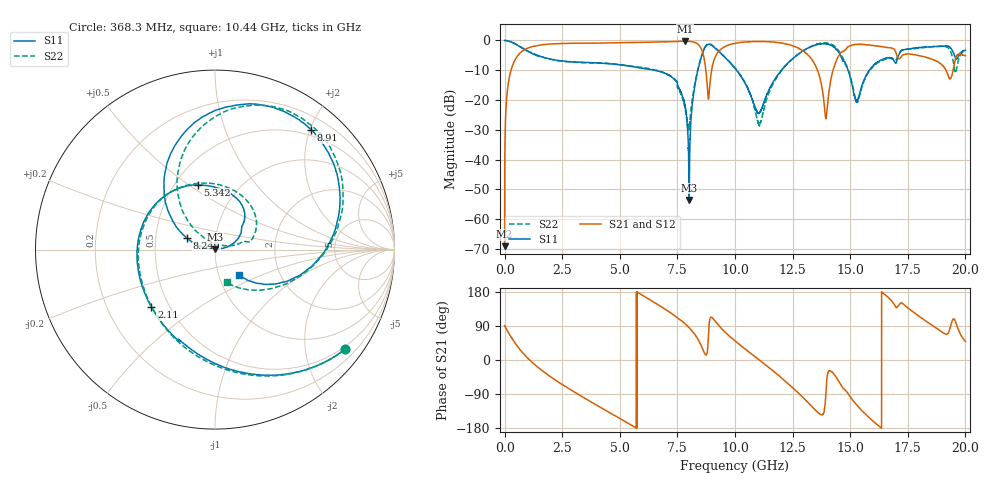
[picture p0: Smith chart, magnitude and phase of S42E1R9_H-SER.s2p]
!{S42E1R9}
!Johanson Technology Inc.
!www.johansontechnology.com
!Test Board Conditions:
!Substrate Type  RO4350B
!Substrate Thickness  50 mil
!Substrate Dk  3.66
!TL Type: GCPW
!TL Trace Width  60 mil
!TL Gap  10 mil
!Electrode orientation  Horizontal
!DUT TOPOLOGY	SERIES
!Mounting Pad LxW  14x55 mil
! Created Wed Nov 25 21:37:39 2020
# khz S ma R 50
! 2 Port Network Data from SP1.SP block
! freq  magS11  angS11  magS21  angS21  magS12  angS12  magS22  angS22
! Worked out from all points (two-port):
!   20001 points, 300 kHz to 20 GHz, reference 50 ohm
!   highest |S21| = -0.25 dB at 7.831 GHz (marker M1); lowest = -69.1 dB at 300 kHz (marker M2)
!   |S21| within 3 dB of the highest: 831.7 MHz to 8.56 GHz (7.729 GHz wide, 165 % of centre); 9.344 GHz to 12.91 GHz (3.565 GHz wide, 32 % of centre)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
!   lowest |S11| = -53.6 dB at 8.009 GHz (marker M3), VSWR 1.00, Z = 50 + j0.209 ohm
!   |S11| at or under -10 dB: 6.507 GHz to 8.388 GHz (1.881 GHz wide, 25.3 % of centre); 10.06 GHz to 12.01 GHz (1.949 GHz wide, 17.7 % of centre); 14.91 GHz to 15.83 GHz (926.2 MHz wide, 6.03 % of centre)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
!   |S22| runs from -30.1 to 0.0 dB; largest |S21 - S12| = 0.017
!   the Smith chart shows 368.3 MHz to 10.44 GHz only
!   S11 on the Smith chart (normalised r, x): 368.3 MHz: 0.43, -2.88; 2.11 GHz: 0.40, -0.33; 5.342 GHz: 0.65, +0.54; 8.249 GHz: 0.72, +0.10; 8.91 GHz: 0.40, +2.02; 10.44 GHz: 1.25, -0.36
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300  0.9996 -0.2  0.0003518 90.4  0.0003525 97.4  1 -0.2
117300  0.989 -12.4  0.14 77.3  0.1402 77.3  0.9895 -12.4
368300  0.9124 -37.6  0.4018 52.8  0.4034 52.8  0.9135 -37.5
2110300  0.4775 -137.9  0.8765 -49.0  0.8765 -49.0  0.4705 -140.3
3334300  0.4305 172.3  0.9002 -95.7  0.8997 -95.7  0.4249 175.8
5342300  0.3736 105.1  0.9178 -166.2  0.9193 -166.4  0.3787 102.3
6667300  0.3055 65.2  0.943 145.5  0.9415 145.4  0.3101 47.9
7831300  0.07897 14.0  0.9717 95.6  0.9709 95.8  0.07275 16.6
8009300  0.002095 86.0  0.9644 85.3  0.9643 85.5  0.03485 92.0
8249300  0.169 157.8  0.9285 68.1  0.9291 68.1  0.1833 134.9
8910300  0.8561 51.2  0.1835 108.4  0.184 108.5  0.8727 48.1
1.00003e7  0.3403 -34.6  0.8948 50.4  0.8949 50.6  0.3444 -40.7
1.04383e7  0.1909 -46.4  0.9416 28.9  0.9416 29.0  0.1949 -69.7
1.10723e7  0.0618 11.4  0.961 -1.0  0.9606 -0.8  0.03882 169.4
1.23283e7  0.4276 27.1  0.8522 -63.6  0.8554 -63.3  0.4265 22.1
1.33343e7  0.7969 -30.1  0.4782 -122.7  0.4831 -122.9  0.8035 -41.1
1.39443e7  0.8761 -79.6  0.04894 -88.1  0.04871 -88.4  0.9089 -85.3
1.44743e7  0.6525 -130.4  0.5275 -52.9  0.5284 -53.1  0.6938 -130.4
1.50913e7  0.1741 -158.2  0.84 -104.3  0.8367 -104.2  0.1836 -156.9
1.66673e7  0.5102 -105.9  0.7591 164.5  0.7473 164.5  0.5016 -110.9
1.83873e7  0.7791 -167.2  0.5091 98.5  0.5119 99.2  0.7766 -177.4
2e7  0.6884 146.9  0.5533 48.9  0.5558 49.8  0.6641 137.5
